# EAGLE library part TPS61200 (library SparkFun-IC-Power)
DC to DC Booster IC-10035
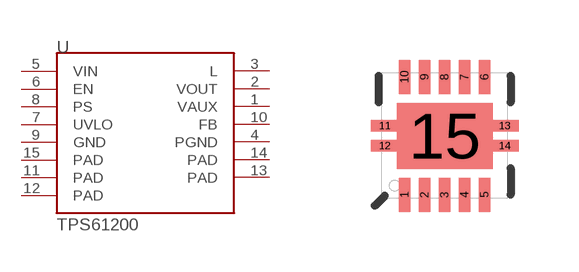
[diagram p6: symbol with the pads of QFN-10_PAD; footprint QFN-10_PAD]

Designator prefix U

## TPS61200 (PROD_ID: IC-10035)  [QFN-10_PAD]
1  VAUX  pas
2  VOUT  pas
3  L  pas
4  PGND  sup
5  VIN  sup
6  EN  in
7  UVLO  pas
8  PS  in
9  GND  sup
10  FB  pas
11  PAD  sup
12  PAD  sup
13  PAD  sup
14  PAD  sup
15  PAD  sup

## Footprint QFN-10_PAD (pad centres in mm)
smd 0.297 x 0.85: 1 -1,-1.475; 2 -0.5,-1.475; 3 0,-1.475; 4 0.5,-1.475; 5 1,-1.475; 6 1,1.475; 7 0.5,1.475; 8 0,1.475; 9 -0.5,1.475; 10 -1,1.475
smd 0.7 x 0.28: 11 -1.5,0.25; 12 -1.5,-0.25; 13 1.5,0.25; 14 1.5,-0.25
smd 2.4 x 1.65: 15 0,0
